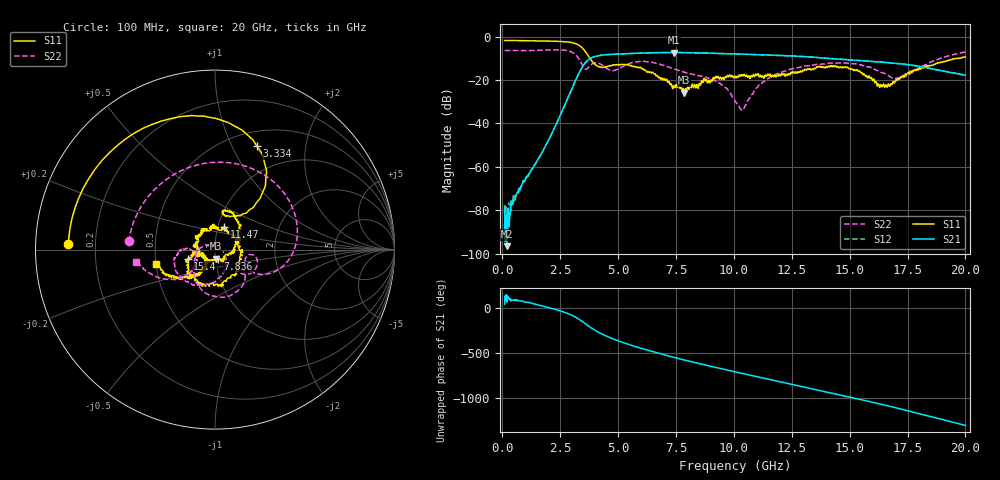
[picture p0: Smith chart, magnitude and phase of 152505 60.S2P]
!  2-Port S-parameters saved by WinCal
! VAR MeasName=S-Parameters (CALIBRATED_DATA) read from VNA (N5230C)
! VAR MeasDate=4/10/2015 9:34:52 AM
! VAR NAME=152505 60
! VAR FILENAME=152505 60.S2P
! VAR DATE=4/10/2015 9:34:52 AM
! VAR PHYS_PORTS=1,2
# Hz S DB R 50
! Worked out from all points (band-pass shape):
!   801 points, 100 MHz to 20 GHz, reference 50 ohm
!   highest |S21| = -7.30 dB at 7.413 GHz (marker M1); lowest = -96.5 dB at 199.5 MHz (marker M2)
!   |S21| within 3 dB of the highest: 3.76 GHz to 14.49 GHz (10.73 GHz wide, 118 % of centre)
!   lowest |S11| = -25.8 dB at 7.861 GHz (marker M3), VSWR 1.11, Z = 50 - j5.14 ohm
!   |S11| at or under -10 dB: 3.785 GHz to 19.63 GHz (15.85 GHz wide, 135 % of centre); 19.69207 GHz to 19.72836 GHz (36.29 MHz wide, 0.184 % of centre)
!   |S22| runs from -34.0 to -6.0 dB; largest |S21 - S12| = 0.0052
!   S11 on the Smith chart (normalised r, x): 100 MHz: 0.10, +0.02; 3.334 GHz: 0.67, +1.25; 7.836 GHz: 1.03, -0.11; 11.47 GHz: 1.07, +0.28; 15.4 GHz: 0.73, -0.08; 20 GHz: 0.50, -0.09
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1e8  -1.75 177.6  -78.45 41.3  -77.51 -150.4  -6.36 174.6
1.995e8  -1.76 175.2  -96.53 66.0  -80.73 -6.8  -6.37 169.2
1.891e9  -2.00 132.3  -49.82 11.8  -49.72 11.6  -6.17 78.9
2.7865e9  -2.40 100.0  -29.37 -56.4  -29.39 -56.7  -6.39 18.2
3.33375e9  -4.13 68.1  -16.27 -127.9  -16.34 -127.8  -10.65 -28.1
3.43325e9  -4.99 60.9  -14.35 -145.7  -14.38 -145.6  -12.63 -31.0
4.1795e9  -13.97 65.7  -8.72 87.5  -8.72 87.5  -12.32 -31.7
5.02525e9  -12.95 73.0  -7.99 -6.6  -8.03 -6.7  -14.77 -34.5
5.871e9  -13.99 44.5  -7.62 -78.7  -7.65 -78.4  -11.51 -65.7
6.741625e9  -18.89 13.2  -7.36 -142.8  -7.38 -142.9  -12.56 -108.6
7.41325e9  -22.62 -38.2  -7.30 171.4  -7.32 171.5  -14.91 -129.9
7.836125e9  -25.04 -73.5  -7.38 143.6  -7.36 143.9  -16.34 -140.0
7.861e9  -25.79 -86.6  -7.38 142.0  -7.35 142.3  -16.39 -139.8
8.831125e9  -20.09 -159.5  -7.57 81.6  -7.61 81.6  -19.03 -164.5
1.005e10  -18.25 139.7  -7.95 10.3  -7.98 10.1  -29.68 125.6
1.039825e10  -18.13 119.5  -8.09 -9.5  -8.08 -9.5  -33.71 49.0
1.146788e10  -17.30 68.5  -8.48 -70.6  -8.47 -70.6  -19.31 -54.7
1.338325e10  -14.85 -61.0  -9.46 -179.7  -9.43 -179.3  -13.08 -115.8
1.539812e10  -15.91 -161.7  -10.95 66.0  -10.95 65.6  -12.69 -168.6
1.669162e10  -22.01 -128.0  -12.01 -11.4  -12.00 -11.8  -18.07 -177.4
1.793538e10  -15.13 -124.0  -13.51 -92.0  -13.64 -92.0  -14.84 -138.0
2e10  -9.38 -166.1  -17.80 132.9  -17.78 133.2  -7.05 -171.1
